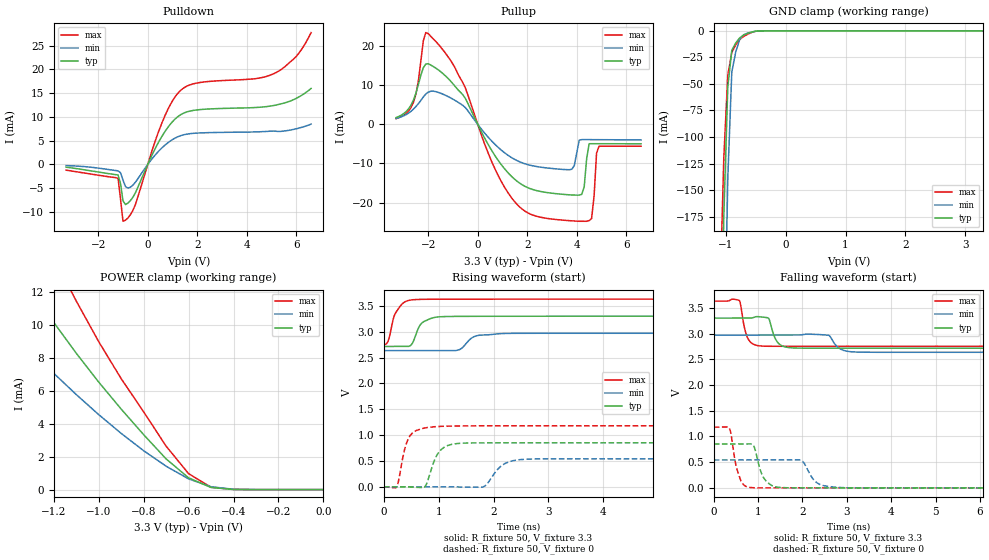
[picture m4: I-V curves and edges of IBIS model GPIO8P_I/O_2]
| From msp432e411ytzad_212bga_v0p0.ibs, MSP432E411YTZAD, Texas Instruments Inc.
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|   Model Cell GPIO8P_I/O_2
[Model]   GPIO8P_I/O_2
Model_type   I/O
Polarity   Non-Inverting
Enable   Active-Low
Vinl =  0.8
Vinh =  2
Cref =  15.0000pF
Rref =  100.0000M
Vref =  0V
Vmeas =  1.65
C_comp   5.378567p   4.597605p   6.118031p
[Model Spec]
Vinl   0.8   0.8   0.8
Vinh   2   2   2
[Temperature Range]   25   125   -40
[Voltage Range]   3.3   2.97   3.63
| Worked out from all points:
|   slope of the pulldown table from 0 to 0.495 V, typ, clamps not added: 95.1 ohm
|   slope of the pullup table from 0 to 0.495 V, typ, clamps not added: 83.2 ohm
|   GND clamp passes 1 mA (typ) near -0.55 V on its own axis
|   POWER clamp passes 1 mA (typ) near -0.62 V on its own axis
|   rising waveform, R_fixture 50, V_fixture 3.3: 20-80 % time 164ps typ, 198ps min, 163ps max; typ from 2.71 V to 3.3 V
|   rising waveform, R_fixture 50, V_fixture 0: 20-80 % time 195ps typ, 262ps min, 164ps max; typ from 0 V to 0.852 V
|   falling waveform, R_fixture 50, V_fixture 3.3: 20-80 % time 155ps typ, 200ps min, 132ps max; typ from 3.3 V to 2.71 V
|   falling waveform, R_fixture 50, V_fixture 0: 20-80 % time 194ps typ, 243ps min, 163ps max; typ from 0.852 V to 0 V
| Nom Voltages:
|   VBAT=3.3, VDDC=1.2, VDD=3.3, GND=0
| Min Voltages:
|   VBAT=2.97, VDDC=1.08, VDD=2.97, GND=0
| Max Voltages:
|   VBAT=3.63, VDDC=1.32, VDD=3.63, GND=0
[POWER_clamp]
|   voltage   I(typ)   I(min)   I(max)
-3.3V     116.1mA    496.8mA    244.3mA
-1.533V   17.14mA    11.87mA    23.97mA
-1.3V     12.14mA    8.433mA    16.92mA
-1.267V   11.48mA    7.98mA     15.99mA
-1.133V   8.919mA    6.212mA    12.36mA
-1.1V     8.296mA    5.781mA    11.47mA
-900mV    4.896mA    3.418mA    6.747mA
-800mV    3.341mA    2.365mA    4.729mA
-700mV    1.867mA    1.423mA    2.643mA
-600mV    716.2uA    650.8uA    969.8uA
-500mV    130.1uA    172.8uA    144.6uA
0V        364.7pA    9.133nA    53.42pA
[Pulldown]
|   voltage   I(typ)   I(min)   I(max)
-3.3V     -584.3uA   -253.2uA   -1.21mA
-1.2V     -2.217mA   -1.357mA   -2.921mA
-1.1V     -4.04mA    -1.763mA   -7.282mA
-1V       -7.684mA   -3.315mA   -11.97mA
-900mV    -8.442mA   -4.658mA   -11.73mA
-500mV    -5.974mA   -3.755mA   -8.425mA
600mV     6.131mA    3.613mA    9.08mA
1.3V      10.36mA    5.99mA     15.43mA
2V        11.47mA    6.588mA    17.13mA
5.1V      12.4mA     7.025mA    19.1mA
6V        13.89mA    7.492mA    22.72mA
6.6V      15.98mA    8.476mA    27.73mA
[Pullup]
|   voltage   I(typ)   I(min)   I(max)
-3.3V     1.74mA     1.511mA    1.455mA
-2.6V     6.179mA    3.882mA    5.603mA
-2.1V     15.44mA    7.747mA    23.48mA
-900mV    9.606mA    6.065mA    14.26mA
800mV     -8.978mA   -5.735mA   -12.76mA
2V        -16.13mA   -10.26mA   -22.55mA
3.8V      -18.05mA   -11.48mA   -24.67mA
4.2V      -17.9mA    -3.901mA   -24.78mA
4.5V      -4.951mA   -3.906mA   -24.61mA
4.6V      -4.948mA   -3.908mA   -24.08mA
4.9V      -4.945mA   -3.917mA   -5.598mA
6.6V      -4.975mA   -3.973mA   -5.588mA
[GND_clamp]
|   voltage   I(typ)   I(min)   I(max)
-3.3V     -16.39A    -15.37A    -17.22A
-1.1V     -384.9mA   -635.5mA   -255.1mA
-1.033V   -175.3mA   -338.1mA   -120.1mA
-966.7mV  -53.11mA   -139.3mA   -41.82mA
-900mV    -18.35mA   -38.91mA   -20.36mA
-833.3mV  -11.36mA   -19.64mA   -13.17mA
-766.7mV  -6.568mA   -7.874mA   -8.128mA
-700mV    -3.981mA   -3.622mA   -5.248mA
-500mV    -326.7uA   -386.2uA   -372.4uA
-366.7mV  -15.8uA    -32.57uA   -14.68uA
3.3V      364.7pA    3.701uA    29.32pA
[Ramp]
| variable   typ   min   max
dV/dt_f 0.36846505/0.15788172n 0.21247855/0.20253052n 0.55003453/0.13382806n
dV/dt_r 0.52052121/0.19593651n 0.33112792/0.26452357n 0.72095857/0.16410135n
R_load = 50
[Rising Waveform]
R_fixture = 50
V_fixture = 3.3
V_fixture_min = 2.97
V_fixture_max = 3.63
|   time   V(typ)   V(min)   V(max)
0s        2.714V     2.635V     2.752V
81ps      2.714V     2.635V     2.826V
187.2ps   2.714V     2.635V     3.303V
284.6ps   2.714V     2.635V     3.474V
490.4ps   2.736V     2.635V     3.613V
579.8ps   2.928V     2.635V     3.622V
728.3ps   3.195V     2.635V     3.627V
1.159ns   3.294V     2.635V     3.629V
2.262ns   3.299V     2.967V     3.63V
20.03ns   3.3V       2.97V      3.63V
[Rising Waveform]
R_fixture = 50
V_fixture = 0
V_fixture_min = 0
V_fixture_max = 0
|   time   V(typ)   V(min)   V(max)
0s        0V         0V         0V
237.6ps   0V         0V         4.448mV
378.9ps   0V         0V         722.4mV
446.6ps   -2.543mV   0V         930.8mV
739.3ps   -7.52mV    0V         1.136V
1.023ns   694.3mV    0V         1.169V
1.792ns   849.9mV    -7.957mV   1.18V
2.217ns   850.6mV    455.2mV    1.18V
2.748ns   851mV      539.5mV    1.18V
20.01ns   852.1mV    541.8mV    1.181V
[Falling Waveform]
R_fixture = 50
V_fixture = 3.3
V_fixture_min = 2.97
V_fixture_max = 3.63
|   time   V(typ)   V(min)   V(max)
0s        3.3V       2.97V      3.63V
576.6ps   3.3V       2.97V      3.64V
759.4ps   3.3V       2.97V      2.921V
1.074ns   3.323V     2.97V      2.756V
1.24ns    3.291V     2.97V      2.752V
1.468ns   2.802V     2.97V      2.752V
1.847ns   2.717V     2.97V      2.752V
2.587ns   2.715V     2.967V     2.752V
3.32ns    2.714V     2.637V     2.752V
20.03ns   2.714V     2.635V     2.752V
[Falling Waveform]
R_fixture = 50
V_fixture = 0
V_fixture_min = 0
V_fixture_max = 0
|   time   V(typ)   V(min)   V(max)
0s        852.2mV    541.8mV    1.181V
349.9ps   852.2mV    541.8mV    1.158V
602.9ps   852mV      541.8mV    155.7mV
926.6ps   756mV      541.8mV    0V
1.136ns   179.1mV    541.8mV    0V
1.529ns   6.045mV    541.7mV    0V
1.981ns   0V         529.5mV    0V
2.386ns   0V         68.03mV    0V
3.05ns    0V         0V         0V
20.01ns   0V         0V         0V
